| TEXAS INSTRUMENTS INCORPORATED
| Standard Linear and Logic Group
| IBIS Model of SN74AVC20T245
| 20-BIT DUAL-SUPPLY BUS TRANSCEIVER WITH CONFIGURABLE VOLTAGE
| TRANSLATION AND 3-STATE OUTPUTS
| This file contains package information for the following:
|  TSSOP 56-pin (DGG) package as [Component] AVC20T245_DGG
|  TVSOP 56-pin (DGV) package as [Component] AVC20T245_DGV
|  VFBGA 56-PIN (GQL) package as [Component] AVC20T245_GQL
| This device can be powered at the following Vccs:
|  1.2 volt Vcc
|  1.5 volt Vcc
|  1.8 volt Vcc
|  2.5 volt Vcc
|  3.3 volt Vcc
| This file provides unique models under the [Model Selector] for each Vcc.
| For operation at a specific Vcc, select the appropriate model after each
| [Model Selector] keyword.
[IBIS Ver]   3.2
[Comment char]  |_char
[File Name]   sn74avc20t245.ibs
[File Rev]   1.2 | b_die
[Date]   April 20, 2004
[Source]   Data created from TI-SPICE simulations at TI-SLL.
[Notes]   The following is an IBIS list for the AVC20T245.
   Please contact sllibis@ti.com with questions and
   comments concerning SLL IBIS models.
   - FILE REV HISTORY
   - 1.2 Release of GQL package on 04/20/04
   - Power clamp data deleted as there is no power-clamp diode.
   - GQL package is package preview only at this date.
   - Due to the fact that the Device is 4.6-V Input/Output
   tolarent, the I/O models has some Non-Monotonic Warnings.
[Disclaimer] Property of Texas Instruments Incorporated.  Unauthorized
   reproduction and/or distribution is strictly prohibited.
   This product is protected under copyright law.
   Created  2003, (C) Copyright  2003, Texas Instruments
   Incorporated, All Rights Reserved
   UNLESS THERE IS A SIGNED, WRITTEN AGREEMENT TO THE
   CONTRARY, TEXAS INSTRUMENTS (TI) IS PROVIDING THE IBIS
   MODELS  AND WITHOUT ANY WARRANTY, EXPRESSED OR
   IMPLIED.  TI assumes no liability for:
   1) the accuracy of the IBIS models provided to your
   company;
   2) the proper functioning of these IBIS Models in your
   design or for any resulting applications; or
   3) infringement of patents, copyrights or intellectual
   property rights resulting from your use of these IBIS
   models.
   TI provides IBIS Models as a service to our customers.
   You and your company shall not distribute, sell or give
   these models to anyone else without prior written
   permission from TI.
   TI reserves the right to make changes to our products or
   to discontinue any semiconductor product or service
   without notice, and advises our customers to obtain the
   latest version of relevant information to verify, before
   placing orders, that the information being relied on is
   current.
   Please be aware that your receipt and use of the IBIS
   information provided shall serve as acceptance of these
   terms and conditions.  If you do not accept these terms,
   you should return or destroy the IBIS models and any
   other accompanying information immediately.
| Component AVC20T245_DGG 56-pin TSSOP
[Component]   AVC20T245_DGG
[Manufacturer]   Texas Instruments, Inc.
[Package]
|   typ   min   max
R_pkg   4.500e-02   3.500e-02   6.200e-02
L_pkg   3.324e-09   2.403e-09   5.094e-09
C_pkg   5.640e-13   3.410e-13   9.140e-13
[Pin]   signal_name   model_name   R_pin   L_pin   C_pin
1   1DIR   AVC20T245_DIR   6.200e-02   5.094e-09   8.560e-13
2   1B1   AVC20T245_IO   6.100e-02   4.621e-09   9.020e-13
3   1B2   AVC20T245_IO   6.000e-02   4.316e-09   8.020e-13
4   GND   GND   5.900e-02   3.968e-09   6.980e-13
5   1B3   AVC20T245_IO   5.700e-02   3.716e-09   6.490e-13
6   1B4   AVC20T245_IO   4.200e-02   3.517e-09   6.530e-13
7   VCCB   POWER   4.100e-02   3.160e-09   5.700e-13
8   1B5   AVC20T245_IO   3.900e-02   2.981e-09   4.820e-13
9   1B6   AVC20T245_IO   3.900e-02   2.808e-09   4.470e-13
10   1B7   AVC20T245_IO   3.800e-02   2.715e-09   4.090e-13
11   GND   GND   4.100e-02   2.675e-09   3.910e-13
12   1B8   AVC20T245_IO   3.900e-02   2.536e-09   3.660e-13
13   1B9   AVC20T245_IO   3.900e-02   2.457e-09   3.480e-13
14   1B10   AVC20T245_IO   3.800e-02   2.411e-09   3.530e-13
15   2B1   AVC20T245_IO   3.900e-02   2.456e-09   3.550e-13
16   2B2   AVC20T245_IO   3.900e-02   2.471e-09   3.490e-13
17   2B3   AVC20T245_IO   4.000e-02   2.580e-09   3.700e-13
18   GND   GND   3.800e-02   2.651e-09   3.890e-13
19   2B4   AVC20T245_IO   3.800e-02   2.739e-09   4.110e-13
20   2B5   AVC20T245_IO   3.900e-02   2.838e-09   4.490e-13
21   2B6   AVC20T245_IO   3.800e-02   2.988e-09   4.840e-13
22   VCCB   POWER   3.800e-02   3.104e-09   5.640e-13
23   2B7   AVC20T245_IO   4.000e-02   3.427e-09   6.380e-13
24   2B8   AVC20T245_IO   5.600e-02   3.654e-09   6.410e-13
25   GND   GND   5.700e-02   3.932e-09   7.000e-13
26   2B9   AVC20T245_IO   5.800e-02   4.257e-09   8.060e-13
27   2B10   AVC20T245_IO   5.700e-02   4.580e-09   9.140e-13
28   2DIR   AVC20T245_DIR   5.900e-02   5.038e-09   8.610e-13
29   2NOE   AVC20T245_NOE   6.000e-02   5.058e-09   8.580e-13
30   2A10   AVC20T245_IO   5.600e-02   4.543e-09   9.040e-13
31   2A9   AVC20T245_IO   5.700e-02   4.241e-09   8.020e-13
32   GND   GND   5.900e-02   3.933e-09   6.990e-13
33   2A8   AVC20T245_IO   5.600e-02   3.616e-09   6.370e-13
34   2A7   AVC20T245_IO   3.700e-02   3.368e-09   6.400e-13
35   VCCA   POWER   3.600e-02   3.024e-09   5.630e-13
36   2A6   AVC20T245_IO   3.500e-02   2.876e-09   4.740e-13
37   2A5   AVC20T245_IO   3.500e-02   2.745e-09   4.440e-13
38   2A4   AVC20T245_IO   3.700e-02   2.683e-09   4.050e-13
39   GND   GND   3.800e-02   2.603e-09   3.820e-13
40   2A3   AVC20T245_IO   3.800e-02   2.510e-09   3.620e-13
41   2A2   AVC20T245_IO   3.600e-02   2.412e-09   3.410e-13
42   2A1   AVC20T245_IO   3.800e-02   2.416e-09   3.490e-13
43   1A10   AVC20T245_IO   3.800e-02   2.403e-09   3.490e-13
44   1A9   AVC20T245_IO   3.700e-02   2.429e-09   3.410e-13
45   1A8   AVC20T245_IO   3.600e-02   2.483e-09   3.580e-13
46   GND   GND   3.700e-02   2.614e-09   3.810e-13
47   1A7   AVC20T245_IO   3.500e-02   2.669e-09   4.020e-13
48   1A6   AVC20T245_IO   3.600e-02   2.763e-09   4.420e-13
49   1A5   AVC20T245_IO   3.600e-02   2.942e-09   4.780e-13
50   VCCA   POWER   3.500e-02   3.053e-09   5.640e-13
51   1A4   AVC20T245_IO   3.600e-02   3.408e-09   6.410e-13
52   1A3   AVC20T245_IO   5.800e-02   3.698e-09   6.410e-13
53   GND   GND   5.900e-02   3.974e-09   6.970e-13
54   1A2   AVC20T245_IO   6.100e-02   4.327e-09   8.020e-13
55   1A1   AVC20T245_IO   6.100e-02   4.624e-09   9.050e-13
56   1NOE   AVC20T245_NOE   6.000e-02   5.063e-09   8.580e-13
| Component AVC20T245_DGV 56-pin TVSOP
[Component]   AVC20T245_DGV
[Manufacturer]   Texas Instruments, Inc.
[Package]
|   typ   min   max
R_pkg   6.300e-02   5.000e-02   8.400e-02
L_pkg   2.945e-09   2.394e-09   3.939e-09
C_pkg   3.910e-13   2.710e-13   5.880e-13
[Pin]   signal_name   model_name   R_pin   L_pin   C_pin
1   1DIR   AVC20T245_DIR   6.800e-02   3.933e-09   5.880e-13
2   1B1   AVC20T245_IO   6.800e-02   3.568e-09   5.870e-13
3   1B2   AVC20T245_IO   7.600e-02   3.464e-09   5.150e-13
4   GND   GND   8.400e-02   3.444e-09   4.590e-13
5   1B3   AVC20T245_IO   8.100e-02   3.277e-09   4.270e-13
6   1B4   AVC20T245_IO   7.400e-02   3.136e-09   3.870e-13
7   VCC   POWER   6.900e-02   2.970e-09   4.010e-13
8   1B5   AVC20T245_IO   5.000e-02   2.785e-09   3.790e-13
9   1B6   AVC20T245_IO   5.100e-02   2.685e-09   3.200e-13
10   1B7   AVC20T245_IO   5.300e-02   2.611e-09   3.160e-13
11   GND   GND   5.300e-02   2.495e-09   2.970e-13
12   1B8   AVC20T245_IO   5.300e-02   2.435e-09   2.920e-13
13   1B9   AVC20T245_IO   5.500e-02   2.412e-09   2.850e-13
14   1B10   AVC20T245_IO   5.600e-02   2.401e-09   2.730e-13
15   2B1   AVC20T245_IO   5.500e-02   2.401e-09   2.730e-13
16   2B2   AVC20T245_IO   5.500e-02   2.399e-09   2.840e-13
17   2B3   AVC20T245_IO   5.400e-02   2.406e-09   2.890e-13
18   GND   GND   5.300e-02   2.450e-09   2.930e-13
19   2B4   AVC20T245_IO   5.100e-02   2.544e-09   3.110e-13
20   2B5   AVC20T245_IO   5.100e-02   2.626e-09   3.150e-13
21   2B6   AVC20T245_IO   5.000e-02   2.727e-09   3.690e-13
22   VCC   POWER   6.500e-02   2.903e-09   3.930e-13
23   2B7   AVC20T245_IO   7.500e-02   3.091e-09   3.860e-13
24   2B8   AVC20T245_IO   8.200e-02   3.272e-09   4.280e-13
25   GND   GND   8.200e-02   3.393e-09   4.570e-13
26   2B9   AVC20T245_IO   7.300e-02   3.380e-09   5.080e-13
27   2B10   AVC20T245_IO   7.100e-02   3.577e-09   5.800e-13
28   2DIR   AVC20T245_DIR   6.800e-02   3.937e-09   5.740e-13
29   2NOE   AVC20T245_NOE   6.900e-02   3.923e-09   5.690e-13
30   2A10   AVC20T245_IO   6.400e-02   3.536e-09   5.740e-13
31   2A9   AVC20T245_IO   7.600e-02   3.428e-09   5.170e-13
32   GND   GND   8.100e-02   3.395e-09   4.680e-13
33   2A8   AVC20T245_IO   8.000e-02   3.255e-09   4.310e-13
34   2A7   AVC20T245_IO   7.100e-02   3.064e-09   3.860e-13
35   VCC   POWER   6.100e-02   2.878e-09   3.890e-13
36   2A6   AVC20T245_IO   5.000e-02   2.710e-09   3.630e-13
37   2A5   AVC20T245_IO   5.000e-02   2.606e-09   3.110e-13
38   2A4   AVC20T245_IO   5.200e-02   2.534e-09   3.060e-13
39   GND   GND   5.200e-02   2.439e-09   2.890e-13
40   2A3   AVC20T245_IO   5.300e-02   2.399e-09   2.860e-13
41   2A2   AVC20T245_IO   5.500e-02   2.394e-09   2.820e-13
42   2A1   AVC20T245_IO   5.500e-02   2.398e-09   2.710e-13
43   1A10   AVC20T245_IO   5.600e-02   2.396e-09   2.710e-13
44   1A9   AVC20T245_IO   5.400e-02   2.402e-09   2.830e-13
45   1A8   AVC20T245_IO   5.400e-02   2.423e-09   2.880e-13
46   GND   GND   5.300e-02   2.474e-09   2.920e-13
47   1A7   AVC20T245_IO   5.100e-02   2.569e-09   3.090e-13
48   1A6   AVC20T245_IO   5.100e-02   2.638e-09   3.130e-13
49   1A5   AVC20T245_IO   5.100e-02   2.742e-09   3.660e-13
50   VCC   POWER   6.400e-02   2.917e-09   3.900e-13
51   1A4   AVC20T245_IO   7.400e-02   3.083e-09   3.830e-13
52   1A3   AVC20T245_IO   8.100e-02   3.249e-09   4.300e-13
53   GND   GND   8.300e-02   3.400e-09   4.550e-13
54   1A2   AVC20T245_IO   7.500e-02   3.427e-09   5.050e-13
55   1A1   AVC20T245_IO   7.100e-02   3.585e-09   5.780e-13
56   1NOE   AVC20T245_NOE   6.900e-02   3.939e-09   5.810e-13
|   VFBGA PACKAGE (GQL)
[Component]   AVC20T245_GQL
[manufacturer]   Texas Instruments, Inc.
[Package]
|   typ   min   max
R_pkg   0.065   0.035   0.097
L_pkg   1.952nH   1.000nH   3.191nH
C_pkg   0.283pF   0.162pF   0.434pF
[Pin] signal_name   model_name   R_pin   L_pin   C_pin
A3   1DIR   AVC20T245_DIR   0.036   1.004nH   0.176pF
A2   1B2   AVC20T245_IO   0.04   1.191nH   0.186pF
A1   1B1   AVC20T245_IO   0.047   1.411nH   0.209pF
B3   GND   GND   0.097   3.191nH   0.434pF
B2   1B4   AVC20T245_IO   0.074   2.213nH   0.329pF
B1   1B3   AVC20T245_IO   0.06   1.712nH   0.243pF
C3   VCCB   POWER   0.085   2.691nH   0.368pF
C2   1B6   AVC20T245_IO   0.074   2.16nH   0.315pF
C1   1B5   AVC20T245_IO   0.06   1.666nH   0.247pF
D2   1B8   AVC20T245_IO   0.074   2.121nH   0.313pF
D3   GND   GND   0.091   2.924nH   0.397pF
D1   1B7   AVC20T245_IO   0.06   1.619nH   0.245pF
E2   1B10   AVC20T245_IO   0.069   2.031nH   0.288pF
E1   1B9   AVC20T245_IO   0.06   1.583nH   0.22pF
F1   2B1   AVC20T245_IO   0.06   1.578nH   0.22pF
F2   2B2   AVC20T245_IO   0.069   2.017nH   0.286pF
G1   2B3   AVC20T245_IO   0.06   1.594nH   0.241pF
G3   GND   GND   0.092   2.917nH   0.397pF
G2   2B4   AVC20T245_IO   0.075   2.114nH   0.315pF
H1   2B5   AVC20T245_IO   0.06   1.632nH   0.247pF
H2   2B6   AVC20T245_IO   0.07   2.074nH   0.307pF
H3   VCCB   POWER   0.086   2.664nH   0.365pF
J1   2B7   AVC20T245_IO   0.06   1.689nH   0.249pF
J2   2B8   AVC20T245_IO   0.066   2.152nH   0.332pF
J3   GND   GND   0.087   3.118nH   0.423pF
K1   2B9   AVC20T245_IO   0.038   1.303nH   0.2pF
K2   2B10   AVC20T245_IO   0.035   1.176nH   0.183pF
K3   2DIR   AVC20T245_DIR   0.035   1.007nH   0.162pF
K4   2NOE   AVC20T245_NOE   0.035   1nH   0.162pF
K5   2A10   AVC20T245_IO   0.035   1.154nH   0.18pF
K6   2A9   AVC20T245_IO   0.041   1.352nH   0.204pF
J4   GND   GND   0.088   3.137nH   0.43pF
J5   2A8   AVC20T245_IO   0.074   2.218nH   0.334pF
J6   2A7   AVC20T245_IO   0.06   1.683nH   0.25pF
H4   VCCA   POWER   0.085   2.658nH   0.372pF
H5   2A6   AVC20T245_IO   0.075   2.149nH   0.321pF
H6   2A5   AVC20T245_IO   0.06   1.627nH   0.248pF
G5   2A4   AVC20T245_IO   0.075   2.113nH   0.314pF
G4   GND   GND   0.092   2.922nH   0.396pF
G6   2A3   AVC20T245_IO   0.06   1.594nH   0.242pF
F5   2A2   AVC20T245_IO   0.069   2.016nH   0.288pF
F6   2A1   AVC20T245_IO   0.06   1.58nH   0.221pF
E6   1A9   AVC20T245_IO   0.06   1.582nH   0.22pF
E5   1A10   AVC20T245_IO   0.069   2.026nH   0.289pF
D6   1A7   AVC20T245_IO   0.06   1.61nH   0.245pF
D4   GND   GND   0.092   2.933nH   0.396pF
D5   1A8   AVC20T245_IO   0.075   2.126nH   0.311pF
C6   1A5   AVC20T245_IO   0.06   1.641nH   0.245pF
C5   1A6   AVC20T245_IO   0.073   2.168nH   0.319pF
C4   VCCA   POWER   0.086   2.675nH   0.362pF
B6   1A3   AVC20T245_IO   0.06   1.688nH   0.243pF
B5   1A4   AVC20T245_IO   0.075   2.281nH   0.333pF
B4   GND   GND   0.095   3.168nH   0.424pF
A6   1A1   AVC20T245_IO   0.045   1.418nH   0.209pF
A5   1A2   AVC20T245_IO   0.039   1.216nH   0.19pF
A4   1NOE   AVC20T245_NOE   0.037   1.029nH   0.179pF
| Model AVC20T245_DIR
[Model Selector]   AVC20T245_DIR
AVC20T245_DIR_12   1.2 volt Vcc
AVC20T245_DIR_15   1.5 volt Vcc
AVC20T245_DIR_18   1.8 volt Vcc
AVC20T245_DIR_25   2.5 volt Vcc
AVC20T245_DIR_33   3.3 volt Vcc
| Model AVC20T245_NOE
[Model Selector]   AVC20T245_NOE
AVC20T245_NOE_12   1.2 volt Vcc
AVC20T245_NOE_15   1.5 volt Vcc
AVC20T245_NOE_18   1.8 volt Vcc
AVC20T245_NOE_25   2.5 volt Vcc
AVC20T245_NOE_33   3.3 volt Vcc
| Model AVC20T245_IO
[Model Selector]   AVC20T245_IO
AVC20T245_IO_12   1.2 volt Vcc
AVC20T245_IO_15   1.5 volt Vcc
AVC20T245_IO_18   1.8 volt Vcc
AVC20T245_IO_25   2.5 volt Vcc
AVC20T245_IO_33   3.3 volt Vcc
| Models and submodels in the file (15): AVC20T245_DIR_12 (Input), AVC20T245_DIR_15 (Input), AVC20T245_DIR_18 (Input), AVC20T245_DIR_25 (Input), AVC20T245_DIR_33 (Input), AVC20T245_NOE_12 (Input), AVC20T245_NOE_15 (Input), AVC20T245_NOE_18 (Input), AVC20T245_NOE_25 (Input), AVC20T245_NOE_33 (Input), AVC20T245_IO_12 (I/O), AVC20T245_IO_15 (I/O), AVC20T245_IO_18 (I/O), AVC20T245_IO_25 (I/O), AVC20T245_IO_33 (I/O)
